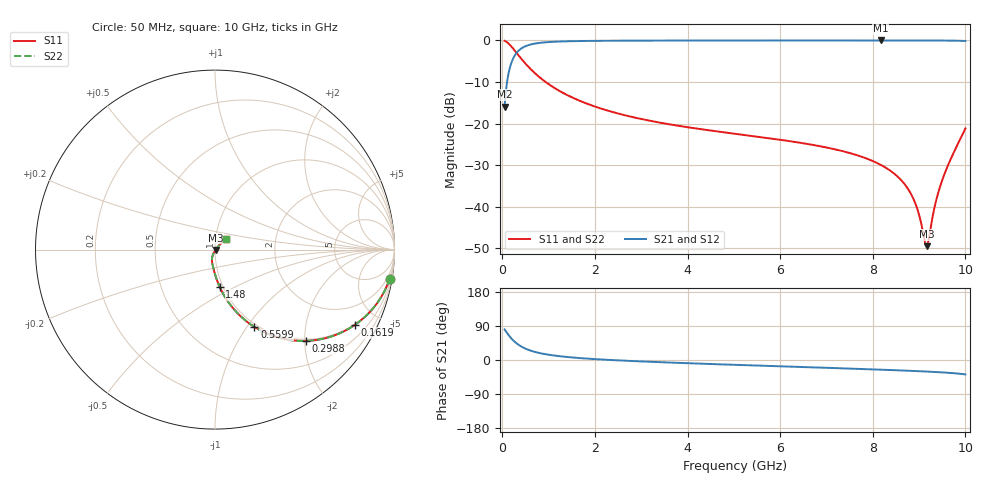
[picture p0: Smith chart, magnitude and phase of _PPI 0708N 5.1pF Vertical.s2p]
! S-Parameter data specifications (vertical orientation):
! Substrate: 40-mil Rogers 3003C, Substrate thickness, H=1.016mm, Dielectric constant, Er=3, Conductor thickness, T_mtl=0.043mm, Loss Tangent, Tand=0.003
! PCB Mounting Pad Footprint: Pad width, PadW=2.54mm , Pad length, PadL=0.51mm , Pad gap, PadG (edge-to-edge)=0.71mm , Reference planes=1.73mm apart
! Created Tue Jan 16 08:45:48 2018
# GHz S MA R 50
! 2 Port Network Data from SP1.SP block
! freq  magS11  angS11  magS21  angS21  magS12  angS12  magS22  angS22
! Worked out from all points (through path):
!   801 points, 50 MHz to 10 GHz, reference 50 ohm
!   highest |S21| = -0.02 dB at 8.172 GHz (marker M1); lowest = -15.9 dB at 50 MHz (marker M2)
!   group delay of S21, straight-line fit = 16.9 ps
!   lowest |S11| = -49.5 dB at 9.167 GHz (marker M3), VSWR 1.01, Z = 50.3 - j0.172 ohm
!   |S11| at or under -10 dB: 935.1 MHz to end of sweep
!   |S22| runs from -49.5 to -0.1 dB; largest |S21 - S12| = 0
!   S11 on the Smith chart (normalised r, x): 50 MHz: 1, -12; 161.9 MHz: 0.96, -3.74; 298.8 MHz: 0.96, -2.03; 559.9 MHz: 0.96, -1.08; 1.48 GHz: 0.96, -0.42; 10 GHz: 1.13, +0.14
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0.05  0.9871 -9.4  0.1602 80.6  0.1602 80.6  0.9871 -9.4
0.1619375  0.8851 -28.3  0.4652 61.7  0.4652 61.7  0.8851 -28.3
0.29875  0.7181 -45.1  0.6956 44.9  0.6956 44.9  0.7181 -45.1
0.423125  0.5893 -55.3  0.8075 34.7  0.8075 34.7  0.5893 -55.3
0.5599375  0.4835 -63.0  0.8749 27.0  0.8749 27.0  0.4835 -63.0
0.9081875  0.3244 -74.1  0.9454 15.8  0.9454 15.8  0.3244 -74.1
1.480312  0.2096 -82.8  0.9771 7.0  0.9771 7.0  0.2096 -82.8
1.716625  0.1835 -85.1  0.9823 4.7  0.9823 4.7  0.1835 -85.1
3.370812  0.1034 -95.1  0.9936 -5.6  0.9936 -5.6  0.1034 -95.1
5.025  0.07544 -101.9  0.9958 -12.8  0.9958 -12.8  0.07544 -101.9
6.691625  0.05562 -107.9  0.9967 -19.4  0.9967 -19.4  0.05562 -107.9
8.171688  0.03193 -111.9  0.9971 -25.5  0.9971 -25.5  0.03193 -111.9
8.345812  0.02795 -111.9  0.9971 -26.3  0.9971 -26.3  0.02795 -111.9
8.619438  0.02073 -110.9  0.997 -27.6  0.997 -27.6  0.02073 -110.9
8.830875  0.01409 -107.7  0.9969 -28.6  0.9969 -28.6  0.01409 -107.7
8.967688  0.009226 -101.0  0.9967 -29.3  0.9967 -29.3  0.009226 -101.0
9.116938  0.004011 -66.5  0.9964 -30.2  0.9964 -30.2  0.004011 -66.5
9.166688  0.003365 -30.6  0.9963 -30.5  0.9963 -30.5  0.003365 -30.6
9.216437  0.00431 4.7  0.9961 -30.8  0.9961 -30.8  0.00431 4.7
9.365687  0.01175 38.1  0.9955 -31.7  0.9955 -31.7  0.01175 38.1
9.490063  0.02017 43.9  0.9947 -32.6  0.9947 -32.6  0.02017 43.9
10  0.08739 43.5  0.983 -38.0  0.983 -38.0  0.08739 43.5
